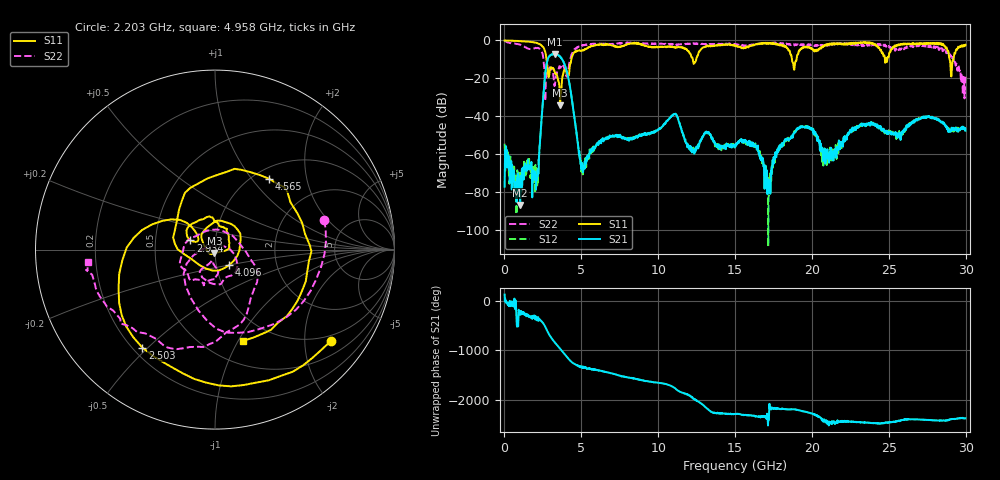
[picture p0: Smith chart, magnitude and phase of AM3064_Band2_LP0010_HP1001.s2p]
# Hz S DB R 50.0
!freq dBS11 angS11 dBS21 angS21 dBS12 angS12 dBS22 angS22
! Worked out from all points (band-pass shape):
!   1600 points, 10 MHz to 29.98 GHz, reference 50 ohm
!   highest |S21| = -7.10 dB at 3.271 GHz (marker M1); lowest = -86.7 dB at 1.022 GHz (marker M2)
!   |S21| within 3 dB of the highest: 2.809 GHz to 3.765 GHz (955.9 MHz wide, 29.1 % of centre)
!   lowest |S11| = -34.1 dB at 3.628 GHz (marker M3), VSWR 1.04, Z = 49.6 - j1.92 ohm
!   |S11| at or under -10 dB: 2.736 GHz to 4.349 GHz (1.613 GHz wide, 45.5 % of centre); 18.7 GHz to 19 GHz (297.5 MHz wide, 1.58 % of centre); 28.95 GHz to 29.2 GHz (253.3 MHz wide, 0.871 % of centre)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
!   |S22| runs from -32.0 to -0.2 dB; largest |S21 - S12| = 0.017
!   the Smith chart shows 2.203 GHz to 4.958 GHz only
!   S11 on the Smith chart (normalised r, x): 2.203 GHz: 0.85, -2.66; 2.503 GHz: 0.24, -0.48; 2.934 GHz: 0.75, +0.08; 4.096 GHz: 1.16, -0.20; 4.565 GHz: 1.18, +1.23; 4.958 GHz: 0.74, -1.05
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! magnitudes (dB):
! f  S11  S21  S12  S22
! 10 MHz  0.0  -77.1  -54.4  -0.2
! 1.022 GHz  -0.4  -86.7  -70.6  -2.3
! 2.203 GHz  -1.7  -70.3  -68.3  -4.0
! 2.503 GHz  -3.3  -31.7  -31.6  -7.9
! 2.934 GHz  -16.7  -8.2  -8.2  -14.4
! 3.271 GHz  -16.6  -7.1  -7.1  -23.7
! 3.628 GHz  -34.1  -8.7  -8.5  -14.2
! 4.096 GHz  -18.6  -17.9  -17.7  -18.8
! 4.565 GHz  -6.1  -41.5  -41.7  -4.5
! 4.958 GHz  -5.5  -65.1  -65.2  -2.9
! 5.015 GHz  -5.5  -68.0  -66.5  -3.0
! 10 GHz  -3.5  -47.1  -46.9  -1.8
! 15 GHz  -2.7  -56.3  -54.8  -1.9
! 16.35 GHz  -2.2  -56.2  -56.0  -2.3
! 17.18 GHz  -1.8  -73.1  -83.2  -1.6
! 17.91 GHz  -2.4  -57.3  -56.3  -1.8
! 19.99 GHz  -4.4  -46.8  -47.1  -2.2
! 21 GHz  -1.9  -57.3  -60.0  -2.8
! 25 GHz  -8.6  -48.2  -47.3  -2.9
! 28.56 GHz  -2.5  -44.0  -43.9  -4.8
! 29.06 GHz  -19.0  -47.7  -47.5  -8.5
! 29.98 GHz  -2.4  -47.6  -47.7  -19.1
